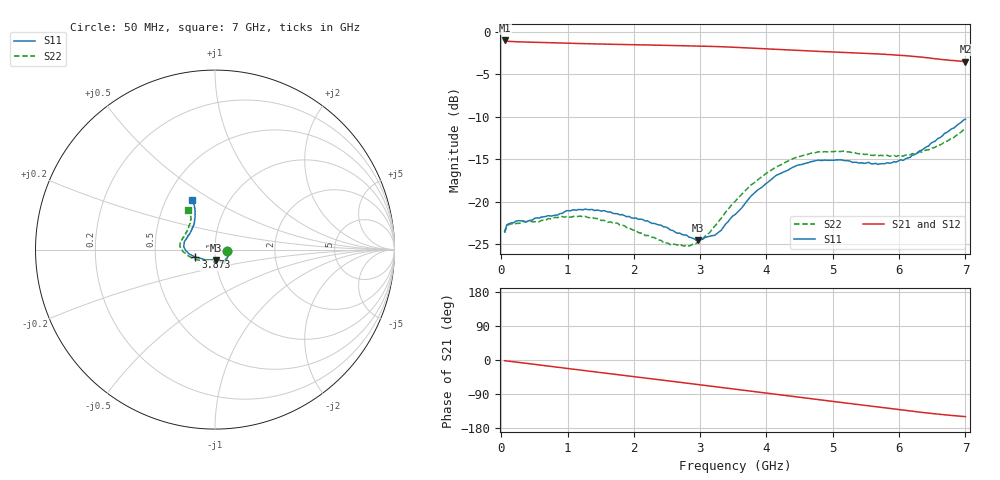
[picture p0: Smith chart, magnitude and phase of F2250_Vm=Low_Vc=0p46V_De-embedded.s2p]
! Integrated Device Technology
! Corporate Headquarters
! 6024 Silver Creek Valley Road
! San Jose, CA 95138  USA
! Phone:  1-408-284-8200
! Toll Free:  1-800-223-1366
! Webpage:  http://www.idt.com/
! Timing and RF Division
! 515 Groton Road, Suite 102
! Westford, MA 01886-6024
! Device:  F2250
! Description: Voltage Variable RF Attenuator
! Frequency:  50.0 -  6000.00 MHz
! Package:  3x3 mm Thin QFN Plastic Package: 16 pin
! Ports:  2 RF, 3 DC
!  Pin  1  = GND
!  Pin  2  = NC
!  Pin  3  = RF1  = Port 1
!  Pin  4  = NC
!  Pin  5  = GND
!  Pin  6  = GND
!  Pin  7  = GND
!  Pin  8  = GND
!  Pin  9  = NC
!  Pin 10  = RF2  = Port 2
!  Pin 11  = NC
!  Pin 12  = GND
!  Pin 13  = GND
!  Pin 14  = VCNTRL
!  Pin 15  = VDD
!  Pin 16  = VMODE
! Vcntrl:  0.460 Volts
! Vmode:  +0.000 Volts
! Vdd:  +3.30  Volts
! Current:  1.127 mA
! Data:  The device was measured on a the F2250 evaluation board which has
!  individual transmission lines to the RF pins.  Data was collected
!  using a calibrated network analyzer.  The evaluation board was
!  de-embedded using a TRL calibration technique.
!  The reference plane is the edge of the package pin.
! Misc:  SN 10
!  Action Tracker AT0258
! Date Measured:  2014-11-26
! Date:  2015-10-15  MJV
! Note:
!  Integrated Device Technology supplies this data as a sample of measured
!  data at the package pin for this product.  Your particular data for this
!  product may vary.
!  Data was taken at 25 degrees C.
!  Integrated Device Technology reserves the right to change this data at anytime.
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# GHz S dB R 50
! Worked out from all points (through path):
!   201 points, 50 MHz to 7 GHz, reference 50 ohm
!   highest |S21| = -1.04 dB at 50 MHz (marker M1); lowest = -3.5 dB at 7 GHz (marker M2)
!   group delay of S21, straight-line fit = 60.1 ps
!   lowest |S11| = -24.5 dB at 2.969 GHz (marker M3), VSWR 1.13, Z = 50 - j5.95 ohm
!   |S11| at or under -10 dB: start of sweep to end of sweep
!   |S22| runs from -25.2 to -11.4 dB; largest |S21 - S12| = 0.00038
!   S11 on the Smith chart (normalised r, x): 50 MHz: 1.14, -0.02; 3.873 GHz: 0.80, -0.07; 7 GHz: 0.67, +0.41
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0.05  -23.51 -8.3  -1.04 -1.8  -1.04 -1.8  -23.67 -9.0
0.08475  -22.71 -8.2  -1.11 -2.5  -1.11 -2.5  -22.83 -8.4
0.15425  -22.48 -10.3  -1.16 -4.0  -1.16 -4.0  -22.60 -10.1
0.71025  -21.64 -34.3  -1.29 -16.2  -1.29 -16.2  -21.98 -36.2
1.2315  -20.96 -51.1  -1.41 -27.4  -1.41 -27.4  -21.78 -56.8
1.75275  -21.42 -57.8  -1.50 -38.5  -1.50 -38.5  -22.51 -65.1
2.37825  -22.73 -59.3  -1.59 -51.8  -1.59 -51.8  -24.50 -69.9
2.552  -23.34 -63.0  -1.61 -55.6  -1.61 -55.6  -25.08 -75.7
2.7605  -23.91 -72.1  -1.65 -60.2  -1.65 -60.2  -25.23 -87.3
2.969  -24.52 -87.0  -1.69 -64.8  -1.69 -64.8  -24.70 -103.6
3.247  -23.79 -115.1  -1.75 -71.0  -1.75 -71.0  -22.63 -126.9
3.525  -21.52 -140.1  -1.84 -77.2  -1.84 -77.2  -19.98 -144.0
3.8725  -18.59 -158.7  -1.97 -84.8  -1.97 -84.8  -17.41 -159.7
4.1505  -16.89 -169.4  -2.08 -90.9  -2.08 -90.9  -15.90 -169.9
4.4285  -15.85 -177.4  -2.19 -96.9  -2.19 -96.9  -14.85 -177.2
4.7065  -15.25 175.7  -2.29 -103.0  -2.29 -103.0  -14.30 176.6
5.15825  -15.12 164.8  -2.45 -112.7  -2.45 -112.7  -14.06 167.2
5.85325  -15.48 141.3  -2.70 -127.6  -2.70 -127.6  -14.65 151.8
6.166  -14.79 130.0  -2.87 -134.4  -2.87 -134.4  -14.49 142.9
6.444  -13.46 121.2  -3.08 -140.2  -3.08 -140.2  -13.91 133.5
6.82625  -11.34 115.1  -3.40 -146.9  -3.40 -146.9  -12.45 125.4
7  -10.28 114.4  -3.52 -149.5  -3.52 -149.5  -11.44 123.9
